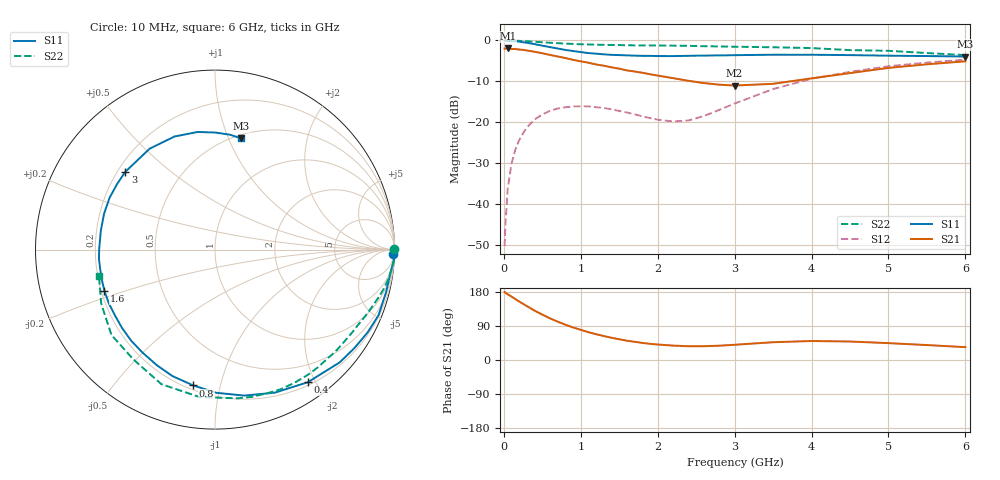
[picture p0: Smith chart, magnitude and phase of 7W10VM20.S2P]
! Infineon Technologies  Discrete & RF Semiconductors
! BFS17W
! Si NPN RF Bipolar Junction Transistor in SOT323
! VCE = 10 V  IC = 0.2 mA
! Common Emitter S-Parameters:  August  1999
# GHz  S  MA  R  50
!  f  S11  S21  S12  S22
! GHz  MAG  ANG  MAG  ANG  MAG  ANG  MAG  ANG
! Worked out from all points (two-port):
!   36 points, 10 MHz to 6 GHz, reference 50 ohm
!   highest |S21| = -1.95 dB at 50 MHz (marker M1); lowest = -11.0 dB at 3 GHz (marker M2)
!   |S21| within 3 dB of the highest: start of sweep to 959.3 MHz
!   lowest |S11| = -3.9 dB at 6 GHz (marker M3), VSWR 4.50, Z = 26.7 + j55.6 ohm
!   |S11| at or under -10 dB: nowhere
!   |S22| runs from -3.6 to 0.0 dB; largest |S21 - S12| = 0.8
!   S11 on the Smith chart (normalised r, x): 10 MHz: 32, -74; 400 MHz: 0.24, -1.90; 800 MHz: 0.23, -0.83; 1.6 GHz: 0.21, -0.17; 3 GHz: 0.23, +0.36; 6 GHz: 0.53, +1.11
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0.01  0.9902 -1.3  0.795 179.5  0.0031 80.5  0.9999 0.2
0.02  0.9993 -3.1  0.795 177.5  0.0056 91.4  0.9996 -0.7
0.05  0.9864 -7.2  0.799 173.5  0.0154 88.3  0.9979 -1.8
0.1  0.9824 -14.0  0.787 167.3  0.0315 81.8  0.9989 -3.6
0.15  0.9818 -21.9  0.786 160.7  0.0467 76.2  0.9926 -5.3
0.25  0.9511 -35.2  0.768 148.2  0.0739 68.2  0.9827 -8.6
0.4  0.902 -55.0  0.728 130.2  0.1089 56.7  0.9641 -13.3
0.6  0.8294 -78.7  0.666 109.9  0.1385 44.2  0.9372 -18.7
0.8  0.7664 -99.1  0.61 93.2  0.1534 34.5  0.9161 -23.8
0.9  0.7435 -108.6  0.58 85.9  0.1567 30.3  0.9065 -26.1
1.1  0.7014 -125.3  0.535 73.3  0.1571 24.2  0.8934 -30.9
1.3  0.6772 -140.0  0.492 63.2  0.1504 20.1  0.8834 -35.8
1.6  0.6577 -159.4  0.431 50.9  0.1321 18.5  0.8737 -43.2
2.2  0.6447 170.7  0.347 38.0  0.1028 38.6  0.8641 -59.1
2.6  0.6545 153.9  0.302 36.4  0.1198 62.3  0.8513 -70.4
3  0.6614 139.1  0.282 40.2  0.1704 73.6  0.8382 -81.3
3.5  0.6698 123.0  0.296 46.9  0.2554 74.1  0.8261 -95.9
4  0.6694 109.7  0.345 50.1  0.3416 68.1  0.8072 -111.7
4.5  0.6625 98.4  0.4 48.8  0.4143 60.2  0.7623 -126.7
5  0.6521 89.7  0.463 44.5  0.485 52.4  0.7477 -140.5
5.5  0.6454 82.5  0.512 39.4  0.5375 44.6  0.7021 -154.6
6  0.6362 76.8  0.557 33.9  0.5827 37.6  0.6628 -167.0
